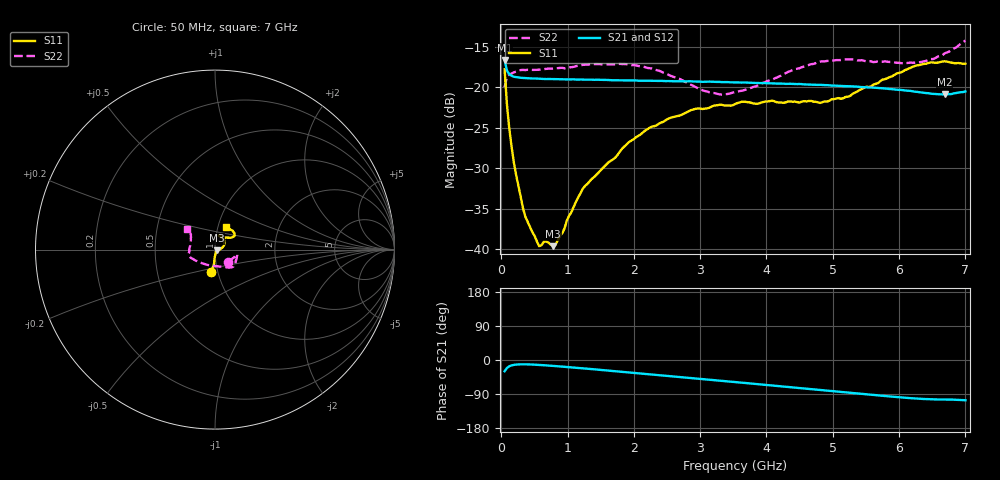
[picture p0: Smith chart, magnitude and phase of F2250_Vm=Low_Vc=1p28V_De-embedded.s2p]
! Integrated Device Technology
! Corporate Headquarters
! 6024 Silver Creek Valley Road
! San Jose, CA 95138  USA
! Phone:  1-408-284-8200
! Toll Free:  1-800-223-1366
! Webpage:  http://www.idt.com/
! Timing and RF Division
! 515 Groton Road, Suite 102
! Westford, MA 01886-6024
! Device:  F2250
! Description: Voltage Variable RF Attenuator
! Frequency:  50.0 -  6000.00 MHz
! Package:  3x3 mm Thin QFN Plastic Package: 16 pin
! Ports:  2 RF, 3 DC
!  Pin  1  = GND
!  Pin  2  = NC
!  Pin  3  = RF1  = Port 1
!  Pin  4  = NC
!  Pin  5  = GND
!  Pin  6  = GND
!  Pin  7  = GND
!  Pin  8  = GND
!  Pin  9  = NC
!  Pin 10  = RF2  = Port 2
!  Pin 11  = NC
!  Pin 12  = GND
!  Pin 13  = GND
!  Pin 14  = VCNTRL
!  Pin 15  = VDD
!  Pin 16  = VMODE
! Vcntrl:  1.280 Volts
! Vmode:  +0.000 Volts
! Vdd:  +3.30  Volts
! Current:  1.192 mA
! Data:  The device was measured on a the F2250 evaluation board which has
!  individual transmission lines to the RF pins.  Data was collected
!  using a calibrated network analyzer.  The evaluation board was
!  de-embedded using a TRL calibration technique.
!  The reference plane is the edge of the package pin.
! Misc:  SN 10
!  Action Tracker AT0258
! Date Measured:  2014-11-26
! Date:  2015-10-15  MJV
! Note:
!  Integrated Device Technology supplies this data as a sample of measured
!  data at the package pin for this product.  Your particular data for this
!  product may vary.
!  Data was taken at 25 degrees C.
!  Integrated Device Technology reserves the right to change this data at anytime.
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# GHz S dB R 50
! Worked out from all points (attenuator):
!   201 points, 50 MHz to 7 GHz, reference 50 ohm
!   highest |S21| = -16.67 dB at 50 MHz (marker M1); lowest = -20.9 dB at 6.687 GHz (marker M2)
!   lowest |S11| = -39.6 dB at 779.8 MHz (marker M3), VSWR 1.02, Z = 51 - j0.454 ohm
!   |S11| at or under -10 dB: start of sweep to end of sweep
!   |S22| runs from -20.9 to -14.2 dB; largest |S21 - S12| = 0.00042
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0.05  -17.80 -99.9  -16.67 -29.7  -16.67 -29.7  -20.02 -42.6
0.08475  -22.11 -93.7  -17.96 -21.1  -17.95 -21.1  -18.72 -20.8
0.15425  -27.33 -92.6  -18.60 -14.3  -18.62 -14.3  -18.33 -13.1
0.22375  -30.84 -86.3  -18.77 -12.1  -18.78 -12.1  -18.09 -12.5
0.328  -34.96 -76.2  -18.87 -11.3  -18.87 -11.3  -17.88 -12.8
0.57125  -39.62 -47.1  -18.97 -13.0  -18.97 -13.0  -17.85 -17.8
0.6755  -39.03 -39.7  -19.01 -14.2  -18.98 -14.2  -17.76 -20.3
0.77975  -39.62 -25.2  -18.99 -15.6  -18.99 -15.5  -17.72 -23.1
0.91875  -38.02 -15.2  -19.04 -17.4  -19.03 -17.4  -17.61 -27.1
1.2315  -32.52 -3.6  -19.08 -21.9  -19.08 -21.9  -17.25 -33.5
1.9265  -26.78 18.1  -19.17 -32.6  -19.17 -32.6  -17.23 -44.4
2.37825  -24.50 29.3  -19.24 -39.7  -19.24 -39.7  -17.96 -52.6
2.86475  -22.83 44.1  -19.28 -47.5  -19.31 -47.5  -19.72 -68.7
3.07325  -22.65 50.7  -19.34 -50.9  -19.34 -50.9  -20.49 -79.7
3.3165  -22.15 58.7  -19.38 -54.8  -19.38 -54.8  -20.92 -95.9
3.525  -22.10 63.3  -19.42 -58.2  -19.42 -58.2  -20.61 -110.5
4.7065  -21.79 67.9  -19.71 -77.5  -19.70 -77.5  -17.14 -159.7
5.22775  -21.19 51.0  -19.88 -86.1  -19.88 -86.1  -16.58 -169.3
5.85325  -18.78 35.9  -20.23 -96.0  -20.23 -96.1  -16.90 177.6
6.33975  -17.21 37.9  -20.66 -102.5  -20.68 -102.5  -16.89 160.2
6.68725  -16.81 46.7  -20.91 -104.3  -20.90 -104.4  -15.84 147.1
7  -17.11 62.8  -20.53 -106.2  -20.56 -106.2  -14.24 144.3
